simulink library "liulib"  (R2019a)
settings: Solver=ode45  StartTime=0.0  StopTime=10.0  RelTol=1e-3  EnableMultiTasking=on
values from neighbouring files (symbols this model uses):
  ag = ones(ng,1); [fPg,fTg] = bfgenD(0,P)    [bfgenD.m]    (also in fbtfit.m = AA \ [Ip ; rBt^2 ; 0]; fbtt.m = zeros(L.ng,1); fgeFpicard.m = x(2+(1:L.ng)))
  aq = []    [fbtt.m]
  aW = []    [fbtt.m]
  D = Fyi1j + Fyim1j + A.*Fyij1  +B.*Fyijm1 - C.*Fyij    [dlst.m]    (also in fbtp.m = meqp(); fgep.m = fgsp(P,varargin{:}))
  dr2FA = dr2Fs(1:nA,1)    [asxycs.m]
  drzFA = drzFs(1:nA,1)    [asxycs.m]
  dz = (z - zx(kz))/dzx    [bintc.m]
  dz2FA = dz2Fs(1:nA,1)    [asxycs.m]
  FA = Fs(1:nA,1)    [asxycs.m]    (also in bfhelp.m = [-1                        0      	 0])
  FB = [0                         1        1]    [bfhelp.m]
  Fx = zeros(n+2,3); Fx(2:end-1,2) = FN    [bfhelp.m]    (also in fbtt.m = meqFx(L,Iy,[Ia;Iu]); fgeFpicard.m = FxP + Fxe)
  FX = Fs(nA+1:ns,1)    [asxycs.m]
  Ie = [Ia;Iu]    [fgeF.m]    (also in fgeFpicard.m = (L.Mee + diag(LXt.dt*L.Re))\       ([LXt.dt*LXt.Va;zeros(L.G)
  IpD = LX.IpD(:,kt)    [fbtt.m]    (also in fgeFpicard.m = LXt.(L.agconc{1,3}))
  Iy = (Iy+flipud(Iy))*0.5    [fbtt.m]    (also in fgeF.m = reshape( xnl(L.ind.iy) , L.nzy, L.nry); fgeFpicard.m = Iyscal*reshape(Tyg*ag,L.nzy,L.nry))
  L = fbtc(P,G)    [fbt.m]    (also in fbtc.m = meqc(P,G,'rrx','zzx'); fbte.m = varargout{1}; fge.m = fgel(L,meqxk(LX,1)); fgec.m = fgsc(P,G))
  lB = false    [fbtt.m]
  lX = false    [fbtt.m]
  nA = numel(rA)    [asxycs.m]    (also in fbtt.m; fgeFpicard.m)
  niter = L.P.itercs    [asxycs.m]    (also in fbtt.m = 2)
  Opy = zeros(meqsize(L, 'Opy'),'int8')    [fbtt.m]
  rA = rs(1:nA,1)    [asxycs.m]    (also in fbtptcv.m = (rA1 + 3*rA2)/4)
  rBt = LX.rBt(kt)    [fbtt.m]    (also in fgeFpicard.m = LXt.rBt)
  rX = rs(nA+1:ns,1)    [asxycs.m]    (also in fbtptcv.m = rzbro(iX,1); fbtxana.m = r0 + [1; 1]*a0*0.5)
  zA = zs(1:nA,1)    [asxycs.m]    (also in fbtptcv.m = (zA1 + 3*zA2)/4)
  zX = zs(nA+1:ns,1)    [asxycs.m]    (also in fbtptcv.m = rzbro(iX,2); fbtxana.m = z0 + [1;-1]*a0*1.0)
undefined symbols (not defined in the file or in its folder): aminor, Bm, bp, bpli2, Brn, Brrn, Brzn, bt, Bzn, Bzrn, Bzzn, delta, deltal, deltau, dzg, epsilon, err, Ff, Fn, Ft, Ft0, FW, Ip, iqQ, iTQ, jtorQ, kappa, li, lp, mu, nX, PpQ, PQ, Q0Q, Q1Q, Q2Q, Q3Q, Q4Q, q95, qmin, raQ, raqmin, rB, rbary, repmat, rgeom, rIp, rIpD, Row, rq, rS, rst, TQ, TTpQ, vector, Vn, Vp, Wk, WN, Wp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
libraries: $bdroot x52, mkllib x48, simulink x7
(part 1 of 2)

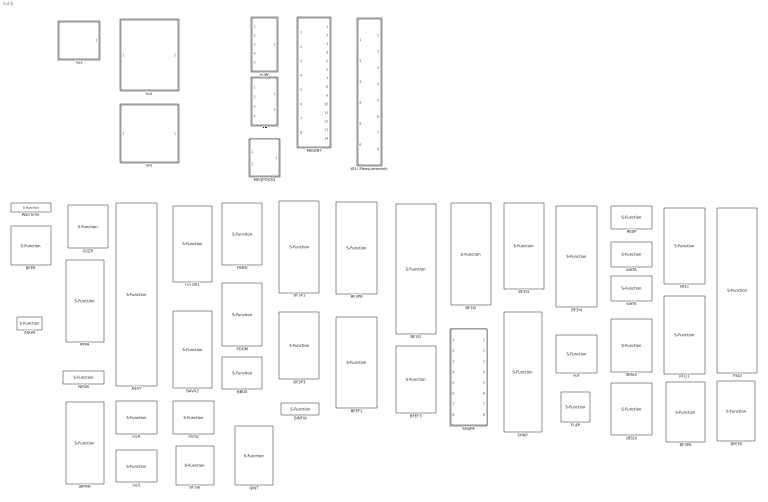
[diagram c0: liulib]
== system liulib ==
  ASGN : S-Function  FunctionName=sasgncsf  Parameters=iu  SFunctionDeploymentMode=off  EnableBusSupport=off  mask{iu=0}
  ASXY : S-Function  FunctionName=sasxycsf  Parameters=rx zx dr dz idr idz Oasx daxm  SFunctionDeploymentMode=off  EnableBusSupport=off  mask{rx=L.G.rx, zx=L.G.zx, dr=L.drx, dz=L.dzx, idr=L.idrx, idz=L.idzx, Oasx=L.Oasx, daxm=L.P.daxm}
      mask prompts: rx "rx [28]"; zx "zx [65]"
      mask help: Axis and Saddle point finder on xy grid
  BAVX2 : S-Function  FunctionName=sbavx2csf  Parameters=a  SFunctionDeploymentMode=off  EnableBusSupport=off  mask{a=0}
      mask prompts: a "alpha"
  BBOX : S-Function  FunctionName=sbboxcsf  Parameters=z r  SFunctionDeploymentMode=off  EnableBusSupport=off  mask{z=L.zy, r=L.ry}
  BF3I1 : S-Function  FunctionName=sbf3i1csf  Parameters=r ir nz nr  SFunctionDeploymentMode=off  EnableBusSupport=off  mask{r=L.ry, ir=L.iry, nz=L.nzy, nr=L.nry}
      mask prompts: r "r inner grid"; ir "ir inner grid"; nz "nzy"; nr "nry"
  BF3I2 : S-Function  FunctionName=sbf3i2csf  SFunctionDeploymentMode=off  EnableBusSupport=off
  BF3I3 : S-Function  FunctionName=sbf3i3csf  Parameters=idsx  SFunctionDeploymentMode=off  EnableBusSupport=off  mask{idsx=L.idsx}
  BF3I4 : S-Function  FunctionName=sbf3i4csf  Parameters=nzy nry  SFunctionDeploymentMode=off  EnableBusSupport=off  mask{nzy=L.nzy, nry=L.nry}
  BF3I6 : S-Function  FunctionName=sbf3i6csf  SFunctionDeploymentMode=off  EnableBusSupport=off
  BF3P1 : S-Function  FunctionName=sbf3p1csf  Parameters=ry iry nzy nry  SFunctionDeploymentMode=off  EnableBusSupport=off  mask{ry=L.ry, iry=L.iry, nzy=L.nzy, nry=L.nry}
      mask prompts: ry "ry inner grid"; iry "iry inner grid"
  BF3P3 : S-Function  FunctionName=sbf3p3csf  Parameters=idsx  SFunctionDeploymentMode=off  EnableBusSupport=off  mask{idsx=L.idsx}
  BF3P6 : S-Function  FunctionName=sbf3p6csf  SFunctionDeploymentMode=off  EnableBusSupport=off
  BF3P8 : S-Function  FunctionName=sbf3p8csf  Parameters=ids iry  SFunctionDeploymentMode=off  EnableBusSupport=off  mask{ids=L.idsx, iry=L.iry}
      mask prompts: ids "r inner grid"; iry "ir inner grid"
  BFEF1 : S-Function  FunctionName=sbfef1csf  Parameters=ry iry nzy nry nP nT  SFunctionDeploymentMode=off  EnableBusSupport=off  mask{ry=L.ry, iry=L.iry, nzy=L.nzy, nry=L.nry, nP=L.P.bfp(1), nT=L.P.bfp(2)}
      mask prompts: ry "ry inner grid"; iry "iry inner grid"
  BFEF3 : S-Function  FunctionName=sbfef3csf  Parameters=ids nP nT  SFunctionDeploymentMode=off  EnableBusSupport=off  mask{ids=L.idsx, nP=L.P.bfp(1), nT=L.P.bfp(2)}
  BFEF6 : S-Function  FunctionName=sbfef6csf  Parameters=nP nT nq  SFunctionDeploymentMode=off  EnableBusSupport=off  mask{nP=L.P.bfp(1), nT=L.P.bfp(2), nq=L.nq}
  BFPR : S-Function  FunctionName=sbfprcsf  SFunctionDeploymentMode=off  EnableBusSupport=off
  BINTW : S-Function  FunctionName=sbintcsf  Parameters=kxW cWx nzx  SFunctionDeploymentMode=off  EnableBusSupport=off  mask{kxW=L.kxW, cWx=L.cWx, nzx=L.nzx}
  FBND : S-Function  FunctionName=sfbndcsf  Parameters=rl zl  SFunctionDeploymentMode=off  EnableBusSupport=off  mask{rl=L.G.rl, zl=L.G.zl}
  FE : Subsystem  Variant=on
  FL4P : S-Function  FunctionName=sfl4pcsf  Parameters=kl cl nz  SFunctionDeploymentMode=off  EnableBusSupport=off  mask{kl=int32(L.kxl-1), cl=L.clx, nz=L.nzx}
      mask prompts: kl "kl 0-based"; cl "cl [4][]"
  FSGI : S-Function  FunctionName=sfsgicsf  Parameters=idoq  SFunctionDeploymentMode=off  EnableBusSupport=off  mask{idoq=1/L.doq}
      mask help: Flux Surface Geometric Integrals
  GSZR : S-Function  FunctionName=sgszrcsf  Parameters=cx cq cr cs ci co  SFunctionDeploymentMode=off  EnableBusSupport=off  mask{cx=L.cx, cq=L.cq, cr=L.cr, cs=L.cs, ci=L.ci, co=L.co}
      mask help: Grad-Shafranov equation on RZ grid
  IPMH : S-Function  FunctionName=sipmhcsf  Parameters=Ahd Aed Ahe Aeh Ahh uAhh nit  SFunctionDeploymentMode=off  EnableBusSupport=off  mask{Ahd=L.Ahd, Aed=L.Aed, Ahe=L.Ahe, Aeh=L.Aeh, Ahh=L.Ahh, uAhh=L.uAhh, nit=L.P.iterh}
      mask prompts: nit "Maximum iteration #"
  MEQINT : Subsystem
  MEQPOSTQ : Subsystem  TreatAsAtomicUnit=on  VariantControl=liuITERQMODEvariant1
  NFDB : S-Function  FunctionName=snfdbcsf  Parameters=nz nr  SFunctionDeploymentMode=off  EnableBusSupport=off  mask{nz=L.nzx, nr=L.nrx}
  PDOM : S-Function  FunctionName=spdomcsf  SFunctionDeploymentMode=off  EnableBusSupport=off
      mask help: Plasma DOmain finder
  QINT : S-Function  FunctionName=sqintcsf  Parameters=rx zx inM  SFunctionDeploymentMode=off  EnableBusSupport=off  mask{rx=L.rx, zx=L.zx, inM=L.inM}
  RESP : S-Function  FunctionName=srespcsf  Parameters=A B nr ng  SFunctionDeploymentMode=off  EnableBusSupport=off  mask{A=L.Wr.*L.Mry, B=L.P.fdz*(L.Wr.*L.Mdzry), nr=L.nr, ng=L.ng}
      mask prompts: A "Mry"; B "Mdzry"
  RTCI : S-Function  FunctionName=srtcicsf  Parameters=c s da nr nz  SFunctionDeploymentMode=off  EnableBusSupport=off  mask{c=L.cdrq, s=L.cdzq, da=L.drx, nr=L.nrx, nz=L.nzx}
      mask prompts: c "cos(theta)*dr"; s "sin(theta)*dz"; da "delta a max"
      mask help: Real-Time Contour Integration
  RTCI1 : S-Function  FunctionName=srtci1csf  SFunctionDeploymentMode=off  EnableBusSupport=off
  SHAP : S-Function  FunctionName=sshapcsf  Parameters=dr dz npq noq  SFunctionDeploymentMode=off  EnableBusSupport=off  mask(Computes shape parameters from rq,zq contours){dr=L.drx, dz=L.dzx, npq=L.npq, noq=L.noq}
      mask help: See shapmex.c, shap.c
  SHAPE : Subsystem  mask(meqshape){dr=L.drx, dz=L.dzx, npq=L.npq, noq=L.noq}
      mask help: Calculates LCFS shape information. See meqshape.m for details
  Wall time : S-Function  FunctionName=swclkcsf  Parameters=f  SFunctionDeploymentMode=off  EnableBusSupport=off  mask{f=1e6}
      mask prompts: f "Factor (e.g. 1000 for ms)"
  dBSLV : S-Function  FunctionName=dbslvcsf  Parameters=niter  SFunctionDeploymentMode=off  EnableBusSupport=off  mask{niter=L.P.iters}
  dIATA : S-Function  FunctionName=diatacsf  SFunctionDeploymentMode=off  EnableBusSupport=off
  dIPMH : S-Function  FunctionName=dipmhcsf  Parameters=Ahd Aed Ahe Aeh Ahh uAhh nit  SFunctionDeploymentMode=off  EnableBusSupport=off  mask{Ahd=0, Aed=0, Ahe=0, Aeh=0, Ahh=0, uAhh=0, nit=0}
      mask prompts: nit "Maximum iteration #"
  l in OX1 : S-Function  FunctionName=sbavxcsf  Parameters=a  SFunctionDeploymentMode=off  EnableBusSupport=off  mask{a=0}
      mask prompts: a "alpha"
  liht : Subsystem  TreatAsAtomicUnit=on
  liuW : Subsystem  TreatAsAtomicUnit=on
  liut : Subsystem  TreatAsAtomicUnit=on
  liux : Subsystem
  locR : S-Function  FunctionName=slocRcsf  Parameters=nR naR  SFunctionDeploymentMode=off  EnableBusSupport=off  mask{nR=numel(L.P.iqR), naR=1}
  locS : S-Function  FunctionName=slocScsf  SFunctionDeploymentMode=off  EnableBusSupport=off
  minQ : S-Function  FunctionName=sminQcsf  Parameters=nmin  SFunctionDeploymentMode=off  EnableBusSupport=off  mask{nmin=1}
  sBSLV : S-Function  FunctionName=sbslvcsf  Parameters=niter  SFunctionDeploymentMode=off  EnableBusSupport=off  mask{niter=L.P.iters}
  sIATA : S-Function  FunctionName=siatacsf  SFunctionDeploymentMode=off  EnableBusSupport=off
  t01/ Measurements : Subsystem
  vizr : S-Function  FunctionName=svizrcsf  Parameters=ry iry dr dz nr nz  SFunctionDeploymentMode=off  EnableBusSupport=off  mask{ry=L.ry, iry=L.iry, dr=L.drx, dz=L.dzx, nr=L.nrx, nz=L.nzx}
      mask prompts: ry "r inner grid"; iry "ir inner grid"

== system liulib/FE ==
  Yd : Inport
  Ie : Inport  Port=2
  Ip : Inport  Port=3
  sIp : Inport  Port=4
  FE ipm : Subsystem  VariantControl=liuHFCTMODEvariant2
  FE ipm double : Subsystem  VariantControl=liuHFCTMODEvariant3
  FE lsq : Subsystem  VariantControl=liuHFCTMODEvariant1
  Jh : Outport
  Je : Outport  Port=2

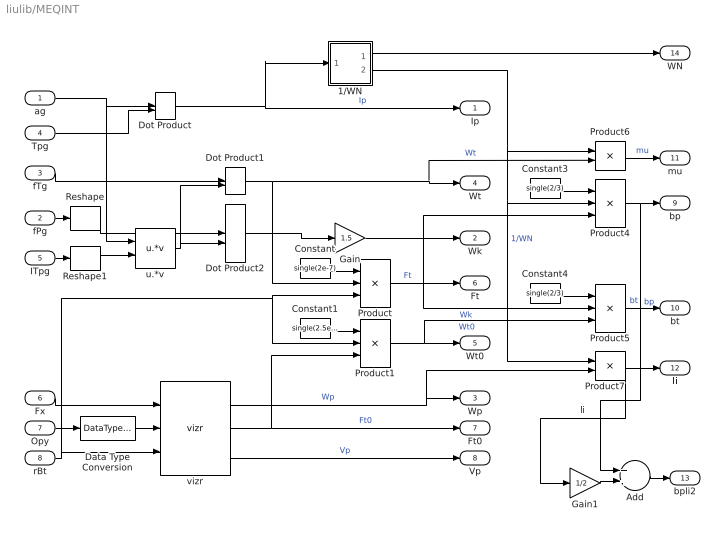
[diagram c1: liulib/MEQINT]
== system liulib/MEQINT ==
  ag : Inport
  fPg : Inport  Port=2
  fTg : Inport  Port=3
  Tpg : Inport  Port=4
  ITpg : Inport  Port=5
  Fx : Inport  Port=6
  Opy : Inport  Port=7
  rBt : Inport  Port=8
  1/WN : Subsystem
  Add : Sum
  Constant : Constant  Value=single(2e-7)  OutDataTypeStr=single
  Constant1 : Constant  Value=single(2.5e6)  OutDataTypeStr=single
  Constant3 : Constant  Value=single(2/3)  OutDataTypeStr=single
  Constant4 : Constant  Value=single(2/3)  OutDataTypeStr=single
  Data Type Conversion : DataTypeConversion  OutDataTypeStr=boolean
  Dot Product : DotProduct
  Dot Product1 : DotProduct
  Dot Product2 : DotProduct
  Gain : Gain  Gain=1.5
  Gain1 : Gain  Gain=1/2
  Product : Product  Inputs=**/
  Product1 : Product  Inputs=3
  Product4 : Product  Inputs=3
  Product5 : Product  Inputs=**/
  Product6 : Product
  Product7 : Product
  Reshape : Reshape
  Reshape1 : Reshape
  u.*v : mkllib/u.*v
  vizr : $bdroot/vizr  ry=L.ry  iry=L.iry  dr=L.drx  dz=L.dzx  nr=L.nrx  nz=L.nzx
  Ip : Outport
  Wk : Outport  Port=2
  Wp : Outport  Port=3
  Wt : Outport  Port=4
  Wt0 : Outport  Port=5
  Ft : Outport  Port=6
  Ft0 : Outport  Port=7
  Vp : Outport  Port=8
  bp : Outport  Port=9
  bt : Outport  Port=10
  mu : Outport  Port=11
  li : Outport  Port=12
  bpli2 : Outport  Port=13
  WN : Outport  Port=14
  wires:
  1/WN/1(WN) -> WN/1
  Gain1/1 -> Add/2
  Add/1 -> bpli2/1
  vizr/3 -> Vp/1  "Vp"
  Fx/1 -> vizr/1
  rBt/1 -> Product1/2, Product/3, vizr/3
  ag/1 -> u.*v/1, Dot Product/1
  Tpg/1 -> Dot Product/2
  u.*v/1 -> Dot Product1/2, Dot Product2/2
  Dot Product/1 -> 1/WN/1(Ip), Ip/1  "Ip"
  Dot Product2/1 -> Gain/1
  vizr/1 -> Product7/2, Wp/1  "Wp"
  Dot Product1/1 -> Product/2, Product6/2, Wt/1  "Wt"
  fTg/1 -> Dot Product1/1
  vizr/2 -> Ft0/1, Product1/3  "Ft0"
  Constant/1 -> Product/1
  Product/1 -> Ft/1  "Ft"
  Constant1/1 -> Product1/1
  Product1/1 -> Product5/3, Wt0/1  "Wt0"
  Constant3/1 -> Product4/1
  Product4/1 -> bp/1, Add/1  "bp"
  Product5/1 -> bt/1  "bt"
  Constant4/1 -> Product5/1
  Product6/1 -> mu/1  "mu"
  Product7/1 -> li/1, Gain1/1  "li"
  Gain/1 -> Product5/2, Product4/3, Wk/1  "Wk"
  1/WN/2(1/WN) -> Product6/1, Product7/1, Product4/2  "1/WN"
  fPg/1 -> Reshape/1
  ITpg/1 -> Reshape1/1
  Reshape/1 -> Dot Product2/1
  Reshape1/1 -> u.*v/2
  Opy/1 -> Data Type Conversion/1
  Data Type Conversion/1 -> vizr/2

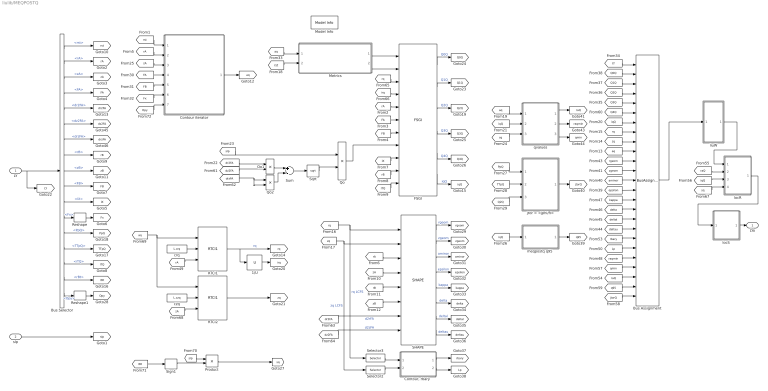
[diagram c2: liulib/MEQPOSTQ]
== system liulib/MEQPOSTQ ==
  LY : Inport
  sIp : Inport  Port=2
  1/U : mkllib/1//U
  Bus Assignment : BusAssignment  AssignedSignals=Q0Q,Q1Q,Q2Q,Q3Q,Q4Q,iqQ,rq,zq,aq,rgeom,zgeom,aminor,epsilon,kappa,delta,deltal,deltau,rbary,lp,raqmin,qmin,raQ,q95,jtorQ
  Bus Selector : BusSelector  OutputSignals=rst,rA,zA,FA,dr2FA,dz2FA,drzFA,rB,zB,FB,lX,Fx,PpQ,TTpQ,iTQ,rBt,Opy
  Contour iterator : Subsystem
  "Contour, rbary " : Subsystem
  FSGI : $bdroot/FSGI  idoq=1/L.doq
  Metrics : Subsystem
  Model Info : simulink/Model-Wide Utilities/Model Info  Frame=on  DisplayStringWithTags=|  HorizontalTextAlignment=Center  LeftAlignmentValue=0.5
      | Model Info
      | %<Creator>
      | %<ModifiedBy>
      | %<ModifiedDate>
      | %<ModifiedComment>
      | %<ModelVersion>
  Product : Product
  Qo : Product  Inputs=**
  Qo1 : Product  Inputs=**
  Qo2 : Product  Inputs=**
  RTCI1 : $bdroot/RTCI1  SFunctionModules=''
  RTCI2 : $bdroot/RTCI1  SFunctionModules=''
  Reshape : Reshape  OutputDimensions=L.nzx*L.nrx
  Reshape1 : Reshape  OutputDimensions=L.nzy*L.nry
  SHAPE : $bdroot/SHAPE  dr=L.drx  dz=L.dzx  npq=L.npq  noq=L.noq
  Selector2 : Selector  NumberOfDimensions=2  InputPortWidth=3  IndexOptions=Select all,Index vector (dialog)  Indices=[1 3],L.npq  OutputSizes=1,1
  Selector3 : Selector  NumberOfDimensions=2  InputPortWidth=3  IndexOptions=Select all,Index vector (dialog)  Indices=[1 3],L.npq  OutputSizes=1,1
  Sign1 : Signum
  Sqrt : Sqrt
  Sum : Sum  Inputs=+-
  crq : Constant  Value=L.crq  OutDataTypeStr=single
  czq : Constant  Value=L.czq  OutDataTypeStr=single
  jtor = <jphi/R> : Subsystem
  liuW : Subsystem  Variant=on  VariantControl=Variant1
  locR : Subsystem  Variant=on  VariantControl=Variant1
  locS : Subsystem  Variant=on  VariantControl=Variant1
  "meqpostq q95 " : Subsystem
  qvalues : Subsystem
  LYo : Outport
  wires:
  "Contour, rbary "/1(rbary) -> [rbary]
  "Contour, rbary "/2(Lp) -> [Lp]
  qvalues/2(raqmin) -> [raqmin]
  qvalues/3(qmin) -> [qmin]
  [iTQ] -> FSGI/11
  FSGI/1 -> [Q0Q]  "Q0Q"
  Bus Selector/5 -> [dr2FA]  "<dr2FA>"
  SHAPE/3 -> [aminor]  "aminor"
  Bus Selector/4 -> [FA]  "<FA>"
  SHAPE/1 -> [rgeom]  "rgeom"
  SHAPE/8 -> [deltau]  "deltau"
  [rq] -> SHAPE/1, Selector3/1  "rq LCFS"
  [sIp] -> Qo/1
  [iqQ] -> qvalues/2(iqQ)
  Selector2/1 -> "Contour, rbary "/2(zq)
  Bus Selector/2 -> [rA]  "<rA>"
  SHAPE/6 -> [delta]  "delta"
  [rB] -> FSGI/10
  Bus Selector/3 -> [zA]  "<zA>"
  FSGI/4 -> [Q3Q]  "Q3Q"
  Sum/1 -> Sqrt/1
  [zq] -> SHAPE/2, Selector2/1  "zq LCFS"
  [FB] -> FSGI/7
  Metrics/1(da^2/pdp = M1q) -> FSGI/1
  FSGI/6 -> [iqQ]  "iqQ"
  Sqrt/1 -> Qo/2
  [dz2FA] -> SHAPE/8  "d2zFA"
  [sq] -> qvalues/3(sq)
  [aq] -> qvalues/1(aq)
  [dr2FA] -> Qo1/1
  [rst] -> Metrics/2(rst)
  [rB] -> SHAPE/5
  FSGI/2 -> [Q1Q]  "Q1Q"
  [zA] -> SHAPE/4
  Qo1/1 -> Sum/1
  Selector3/1 -> "Contour, rbary "/1(rq)
  SHAPE/4 -> [epsilon]  "epsilon"
  SHAPE/2 -> [zgeom]  "zgeom"
  SHAPE/7 -> [deltal]  "deltal"
  [drzFA] -> Qo2/2, Qo2/1
  [rA] -> SHAPE/3
  [rA] -> FSGI/5
  Qo/1 -> FSGI/8
  [FA] -> FSGI/6
  Qo2/1 -> Sum/2
  Metrics/2(((da^2/2do)^2+a^2)/(da^2/pdp) = M2q) -> FSGI/2
  [zB] -> SHAPE/6
  [lX] -> FSGI/9
  [dr2FA] -> SHAPE/7  "d2rFA"
  SHAPE/5 -> [kappa]  "kappa"
  [dz2FA] -> Qo1/2
  sIp/1 -> [sIp]
  FSGI/3 -> [Q2Q]  "Q2Q"
  FSGI/5 -> [Q4Q]  "Q4Q"
  Bus Selector/1 -> [rst]  "<rst>"
  [iqQ] -> "meqpostq q95 "/1(iqQ)
  "meqpostq q95 "/1(q95) -> [q95]
  [PpQ] -> jtor = <jphi/R>/1(PpQ)
  [TTpQ] -> jtor = <jphi/R>/2(TTpQ)
  [Q2Q] -> jtor = <jphi/R>/3(Q2Q)
  jtor = <jphi/R>/1(jtorQ) -> [jtorQ]
  qvalues/1(raQ) -> [raQ]
  [zA] -> Contour iterator/3(zA)
  [FB] -> Contour iterator/5(FB)
  [rst] -> Contour iterator/1(rst)
  [rA] -> Contour iterator/2(rA)
  [FA] -> Contour iterator/4(FA)
  [Fx] -> Contour iterator/6(Fx)
  Contour iterator/1(aq) -> [aq]
  [aq] -> Metrics/1(aq)
  LY/1 -> [LY], Bus Selector/1
  [jtorQ] -> Bus Assignment/25
  [q95] -> Bus Assignment/24
  [Lp] -> Bus Assignment/20
  [rbary] -> Bus Assignment/19
  [deltau] -> Bus Assignment/18
  [deltal] -> Bus Assignment/17
  [delta] -> Bus Assignment/16
  [kappa] -> Bus Assignment/15
  [epsilon] -> Bus Assignment/14
  [aminor] -> Bus Assignment/13
  [zgeom] -> Bus Assignment/12
  [rgeom] -> Bus Assignment/11
  [aq] -> Bus Assignment/10
  [zq] -> Bus Assignment/9
  [rq] -> Bus Assignment/8
  [iqQ] -> Bus Assignment/7
  [Q4Q] -> Bus Assignment/6
  [Q3Q] -> Bus Assignment/5
  [Q2Q] -> Bus Assignment/4
  [Q1Q] -> Bus Assignment/3
  [Q0Q] -> Bus Assignment/2
  [LY] -> Bus Assignment/1
  Bus Selector/6 -> [dz2FA]  "<dz2FA>"
  Bus Selector/7 -> [drzFA]  "<drzFA>"
  Bus Selector/8 -> [rB]  "<rB>"
  Bus Selector/9 -> [zB]  "<zB>"
  Bus Selector/10 -> [FB]  "<FB>"
  Bus Selector/11 -> [lX]  "<lX>"
  Bus Selector/13 -> [PpQ]  "<PpQ>"
  Bus Selector/14 -> [TTpQ]  "<TTpQ>"
  Bus Selector/15 -> [iTQ]  "<iTQ>"
  Reshape/1 -> [Fx]
  Bus Selector/12 -> Reshape/1  "<Fx>"
  [irq] -> FSGI/4
  [rq] -> FSGI/3
  locS/1(" LYo") -> LYo/1
  Bus Assignment/1 -> liuW/1(LY)
  [raQ] -> locR/2("raQ ")
  [iqQ] -> locR/3("qQ ")
  [sq] -> locR/4(sq)
  liuW/1(LYo) -> locR/1(LY)
  locR/1(" LYo") -> locS/1("LY ")
  [raqmin] -> Bus Assignment/21
  [qmin] -> Bus Assignment/22
  [raQ] -> Bus Assignment/23
  RTCI1/1 -> [rq], 1/U/1  "rq"
  crq/1 -> RTCI1/2
  czq/1 -> RTCI2/2
  [zA] -> RTCI2/3
  [aq] -> RTCI2/1, RTCI1/1
  [rA] -> RTCI1/3
  1/U/1 -> [irq]
  RTCI2/1 -> [zq]
  Sign1/1 -> Product/2
  [sIp] -> Product/1
  Product/1 -> [sq]
  Bus Selector/16 -> [rBt]  "<rBt>"
  [rBt] -> Sign1/1
  [Opy] -> Contour iterator/7(Opy)
  Bus Selector/17 -> Reshape1/1  "<Opy>"
  Reshape1/1 -> [Opy]

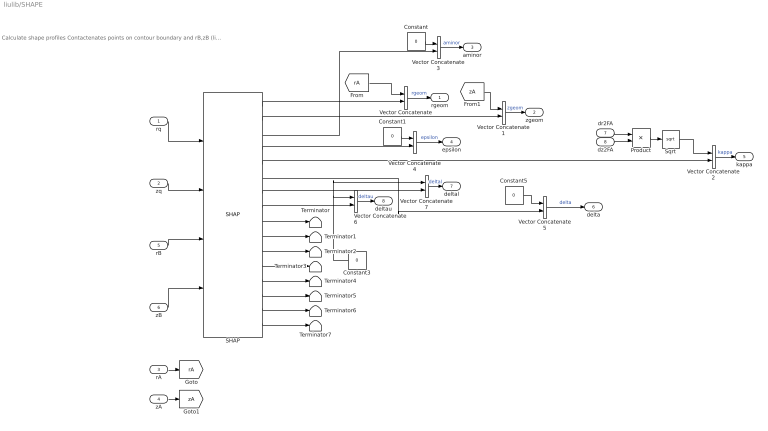
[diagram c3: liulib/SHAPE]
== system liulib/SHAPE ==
  note: Calculate shape profiles Contactenates points on contour boundary and rB,zB (limiter/divertor point) see also meqshape.m
  rq : Inport  OutDataTypeStr=single
  zq : Inport  Port=2  OutDataTypeStr=single
  rA : Inport  Port=3  OutDataTypeStr=single
  zA : Inport  Port=4  OutDataTypeStr=single
  rB : Inport  Port=5  OutDataTypeStr=single
  zB : Inport  Port=6  OutDataTypeStr=single
  dr2FA : Inport  Port=7
  dz2FA : Inport  Port=8
  Constant{,1,3,5} (4 alike) : Constant  Value=0  OutDataTypeStr=single
  Product : Product  Inputs=*/
  SHAP : $bdroot/SHAP  dr=L.drx  dz=L.dzx  npq=L.npq  noq=L.noq
  Sqrt : Sqrt
  Terminator{,1..7} (8 alike) : Terminator
  Vector Concatenate{,1..7} (8 alike) : Concatenate
  rgeom : Outport
  zgeom : Outport  Port=2
  aminor : Outport  Port=3
  epsilon : Outport  Port=4
  kappa : Outport  Port=5
  delta : Outport  Port=6
  deltal : Outport  Port=7
  deltau : Outport  Port=8
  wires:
  SHAP/6 -> Vector Concatenate5/2
  SHAP/4 -> Vector Concatenate4/2
  rq/1 -> SHAP/1
  zq/1 -> SHAP/2
  zB/1 -> SHAP/4
  rB/1 -> SHAP/3
  SHAP/1 -> Vector Concatenate/2
  SHAP/3 -> Vector Concatenate3/2
  SHAP/5 -> Vector Concatenate2/2
  SHAP/7 -> Vector Concatenate7/2
  SHAP/9 -> Terminator/1
  SHAP/8 -> Vector Concatenate6/2
  SHAP/10 -> Terminator1/1
  SHAP/11 -> Terminator2/1
  SHAP/12 -> Terminator3/1
  SHAP/13 -> Terminator4/1
  SHAP/14 -> Terminator5/1
  SHAP/15 -> Terminator6/1
  SHAP/16 -> Terminator7/1
  Vector Concatenate/1 -> rgeom/1  "rgeom"
  rA/1 -> [rA]
  [rA] -> Vector Concatenate/1
  zA/1 -> [zA]
  [zA] -> Vector Concatenate1/1
  SHAP/2 -> Vector Concatenate1/2
  Vector Concatenate1/1 -> zgeom/1  "zgeom"
  Vector Concatenate2/1 -> kappa/1  "kappa"
  Vector Concatenate3/1 -> aminor/1  "aminor"
  Vector Concatenate4/1 -> epsilon/1  "epsilon"
  Constant/1 -> Vector Concatenate3/1
  Constant1/1 -> Vector Concatenate4/1
  Vector Concatenate5/1 -> delta/1  "delta"
  Vector Concatenate6/1 -> deltau/1  "deltau"
  Constant3/1 -> Vector Concatenate7/1, Vector Concatenate6/1
  Vector Concatenate7/1 -> deltal/1  "deltal"
  Constant5/1 -> Vector Concatenate5/1
  Product/1 -> Sqrt/1
  Sqrt/1 -> Vector Concatenate2/1
  dz2FA/1 -> Product/2
  dr2FA/1 -> Product/1

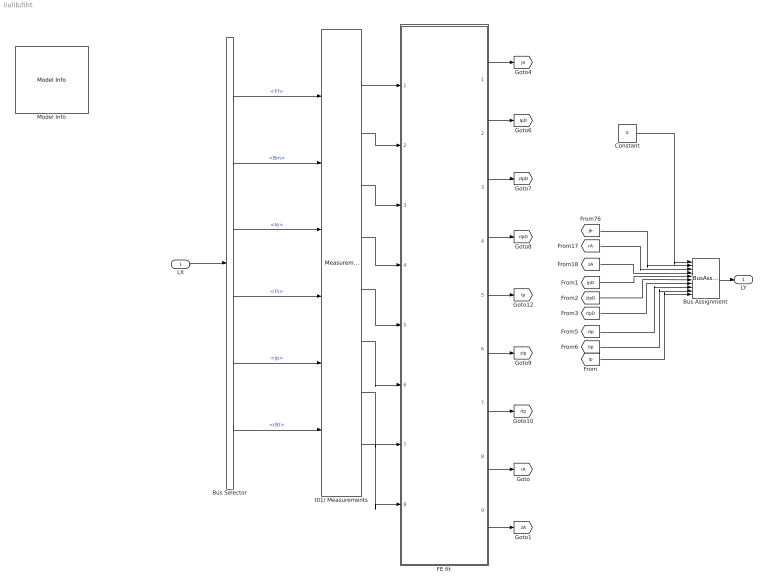
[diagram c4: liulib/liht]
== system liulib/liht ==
  LX : Inport
  Bus Assignment : BusAssignment  AssignedSignals=Ie,rA,zA,IpD,zIpD,rIpD,zIp,rIp,Ip
  Bus Selector : BusSelector  OutputSignals=Ff,Bm,Ie,Ft,Ip,rBt
  Constant : Constant  Value=0  OutDataTypeStr=Bus: LYbus
  FE fit : Subsystem
  Model Info : simulink/Model-Wide Utilities/Model Info  Frame=on  DisplayStringWithTags=|  HorizontalTextAlignment=Center  LeftAlignmentValue=0.5
      | Model Info
      | %<Creator>
      | %<ModifiedBy>
      | %<ModifiedDate>
      | %<ModifiedComment>
      | %<ModelVersion>
  t01/ Measurements : $bdroot/t01// Measurements  SystemSampleTime=-1
  LY : Outport
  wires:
  FE fit/6(Out7) -> [zIp]
  FE fit/7(Out8) -> [rIp]
  FE fit/5(Out9) -> [Ip]
  FE fit/8(Out5) -> [rA]
  [Ip] -> Bus Assignment/10
  [rIp] -> Bus Assignment/9
  [zIp] -> Bus Assignment/8
  Bus Assignment/1 -> LY/1
  Bus Selector/6 -> t01/ Measurements/6  "<rBt>"
  Bus Selector/4 -> t01/ Measurements/4  "<Ft>"
  t01/ Measurements/4 -> FE fit/4(Ie)
  Bus Selector/3 -> t01/ Measurements/3  "<Ie>"
  Bus Selector/5 -> t01/ Measurements/5  "<Ip>"
  LX/1 -> Bus Selector/1
  t01/ Measurements/8 -> FE fit/8(sIp)
  t01/ Measurements/7 -> FE fit/7(FN)
  t01/ Measurements/6 -> FE fit/6(rBt)
  t01/ Measurements/5 -> FE fit/5(Ip)
  t01/ Measurements/3 -> FE fit/3(Yi)
  t01/ Measurements/2 -> FE fit/2(Yd)
  Bus Selector/1 -> t01/ Measurements/1  "<Ff>"
  Bus Selector/2 -> t01/ Measurements/2  "<Bm>"
  t01/ Measurements/1 -> FE fit/1(Yr)
  FE fit/1(Out4) -> [Je]
  FE fit/9(Out6) -> [zA]
  FE fit/2(Out1) -> [IpD]
  FE fit/3(Out2) -> [zIpD]
  FE fit/4(Out3) -> [rIpD]
  Constant/1 -> Bus Assignment/1
  [Je] -> Bus Assignment/2
  [IpD] -> Bus Assignment/5
  [zIpD] -> Bus Assignment/6
  [rIpD] -> Bus Assignment/7
  [rA] -> Bus Assignment/3
  [zA] -> Bus Assignment/4

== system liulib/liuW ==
  zaW : Inport
  rst : Inport  Port=2
  FW : Inport  Port=3
  Fx : Inport  Port=4
  Opy : Inport  Port=5
  BINTW : $bdroot/BINTW  kxW=L.kxW  cWx=L.cWx  nzx=L.nzx
  Constant : Constant  Value=int8(0)
  IC = 1 : UnitDelay  InitialCondition=1  SampleTime=-1  HasFrameUpgradeWarning=on
  RTCI : $bdroot/RTCI  c=L.cdrW  s=L.cdzW  da=L.drx  nr=L.nrx  nz=L.nzx
  Reshape1 : Reshape
  Reshape2 : Reshape
  "aq " : Switch  Criteria=u2 ~= 0
  dan : Terminator
  rx1 : Constant  Value=L.erW  OutDataTypeStr=single
  rx2 : Constant  Value=L.ezW  OutDataTypeStr=single
  rx3 : Constant  Value=zeros(L.G.nW,L.P.nFW)  VectorParams1D=off  OutDataTypeStr=single
  aW : Outport
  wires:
  Reshape2/1 -> RTCI/6
  Reshape1/1 -> BINTW/1, RTCI/4
  rst/1 -> IC = 1/1
  zaW/1 -> "aq "/3
  FW/1 -> RTCI/5
  "aq "/1 -> RTCI/1
  RTCI/2 -> dan/1
  rx1/1 -> RTCI/2
  rx2/1 -> RTCI/3
  Fx/1 -> Reshape1/1
  rx3/1 -> "aq "/1
  RTCI/1 -> aW/1  "aW"
  BINTW/1 -> RTCI/7
  Constant/1 -> RTCI/8
  Opy/1 -> Reshape2/1
  IC = 1/1 -> "aq "/2

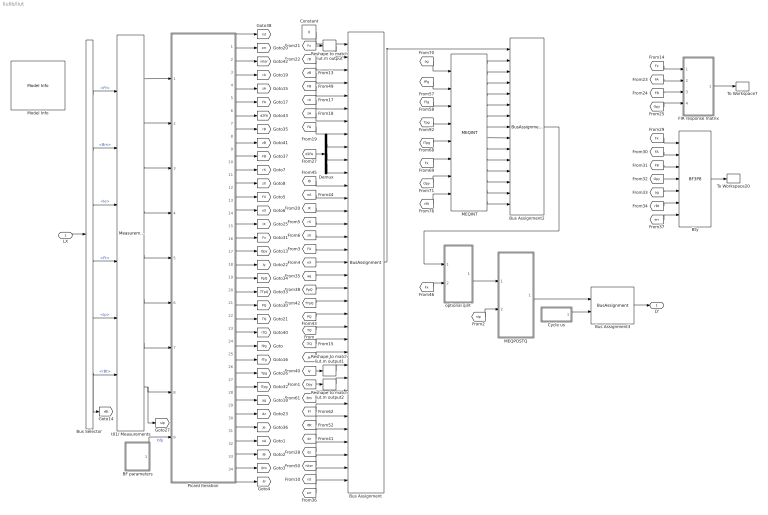
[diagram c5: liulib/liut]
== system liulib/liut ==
  LX : Inport
  BF parameters : Subsystem  Variant=on  VariantControl=Variant1
  Bty : $bdroot/BF3P8  Commented=on  ids=L.idsx  iry=L.iry
  Bus Assignment : BusAssignment  AssignedSignals=Fx,rB,zB,FB,rA,zA,FA,dr2FA,dz2FA,drzFA,lB,nA,lX,rX,zX,FX,nX,ag,PpQ,TTpQ,PQ,TQ,iTQ,Ie,Iy,Opy,Bm,Ff,rBt,dz,dzg,niter,rst,err
  Bus Assignment2 : BusAssignment  AssignedSignals=Ip,Wk,Wp,Wt,Wt0,Ft,Ft0,Vp,bp,bt,mu,li,bpli2,WN
  Bus Assignment3 : BusAssignment  AssignedSignals=cycle
  Bus Selector : BusSelector  OutputSignals=Ff,Bm,Ie,Ft,Ip,rBt
  Constant : Constant  Value=0  OutDataTypeStr=Bus: LYbus
  Cycle us : Subsystem
  Demux : Demux  Outputs=3
  FIR response matrix : Subsystem  Commented=on
  MEQINT : $bdroot/MEQINT  SystemSampleTime=-1
  MEQPOSTQ : Subsystem  Variant=on  VariantControl=Variant1
  Model Info : simulink/Model-Wide Utilities/Model Info  Frame=on  DisplayStringWithTags=|  HorizontalTextAlignment=Center  LeftAlignmentValue=0.5
      | Model Info
      | %<Creator>
      | %<ModifiedBy>
      | %<ModifiedDate>
      | %<ModifiedComment>
      | %<ModelVersion>
  Picard Iteration : Subsystem
  Reshape to match liut.m output : Reshape  OutputDimensionality=Customize  OutputDimensions=[L.nzx,L.nrx]
  Reshape to match liut.m output1 : Reshape  OutputDimensionality=Customize  OutputDimensions=[L.nzy,L.nry]
  Reshape to match liut.m output2 : Reshape  OutputDimensionality=Customize  OutputDimensions=[L.nzy,L.nry]
  To Workspace20 : ToWorkspace  VariableName=Bty  SampleTime=-1
  To Workspace7 : ToWorkspace  VariableName=Tdg  SampleTime=-1
  optional qint : Subsystem  Variant=on  VariantControl=Variant1
  t01/ Measurements : $bdroot/t01// Measurements  SystemSampleTime=-1
  LY : Outport
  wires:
  [zX] -> Bus Assignment/16
  [rX] -> Bus Assignment/15
  Picard Iteration/12(Out34) -> [zX]
  Picard Iteration/11(Out33) -> [rX]
  [nX] -> Bus Assignment/18
  Picard Iteration/14(Out32) -> [nX]
  [FX] -> Bus Assignment/17
  Bus Assignment2/1 -> optional qint/1("LY ")
  [Fx] -> optional qint/2(Fx)
  Picard Iteration/34(Out30) -> [Ff]
  Picard Iteration/33(Out29) -> [Bm]
  MEQINT/14 -> Bus Assignment2/15
  [iTQ] -> Bus Assignment/24
  Reshape to match liut.m output1/1 -> Bus Assignment/26
  [Iy] -> Reshape to match liut.m output1/1
  [Je] -> Bus Assignment/25
  Bus Selector/6 -> t01/ Measurements/6, [rBt]  "<rBt>"
  Bus Selector/4 -> t01/ Measurements/4  "<Ft>"
  [Opy] -> FIR response matrix/4(Opy)
  [FA] -> Bty/2
  [FA] -> FIR response matrix/2(FA)
  FIR response matrix/1(Tdg) -> To Workspace7/1
  [Opy] -> Bty/4
  [rBt] -> Bty/6
  Bty/1 -> To Workspace20/1
  [Fx] -> FIR response matrix/1(Fx)
  [ag] -> Bty/5
  [FB] -> FIR response matrix/3(FB)
  [Fx] -> Bty/1
  [FB] -> Bty/3
  [err] -> Bty/7
  Bus Assignment3/1 -> LY/1
  Cycle us/1(Out1) -> Bus Assignment3/2
  Reshape to match liut.m output/1 -> Bus Assignment/2
  MEQINT/13 -> Bus Assignment2/14
  Bus Assignment/1 -> Bus Assignment2/1
  [TQ] -> Bus Assignment/23
  [PQ] -> Bus Assignment/22
  [TTpQ] -> Bus Assignment/21
  [PpQ] -> Bus Assignment/20
  [lX] -> Bus Assignment/14
  [ag] -> Bus Assignment/19
  [nA] -> Bus Assignment/13
  [lB] -> Bus Assignment/12
  Picard Iteration/32(Out28) -> [lB]
  Picard Iteration/31(Out27) -> [nA]
  [Fx] -> Reshape to match liut.m output/1
  [rB] -> Bus Assignment/3
  [zB] -> Bus Assignment/4
  [FB] -> Bus Assignment/5
  [d2FA] -> Demux/1
  Demux/2 -> Bus Assignment/10
  Demux/3 -> Bus Assignment/11
  Demux/1 -> Bus Assignment/9
  [FA] -> Bus Assignment/8
  [zA] -> Bus Assignment/7
  [rA] -> Bus Assignment/6
  Picard Iteration/23(Out18) -> [iTQ]
  Picard Iteration/19(Out25) -> [PpQ]
  Picard Iteration/29(Out24) -> [dz]
  Picard Iteration/18(Out15) -> [Iy]
  Picard Iteration/5(Out6) -> [zA]
  Picard Iteration/30(Out4) -> [Je]
  Picard Iteration/20(Out26) -> [TTpQ]
  Picard Iteration/10(Out11) -> [FB]
  Picard Iteration/27(Out22) -> [ITpg]
  Picard Iteration/22(Out17) -> [TQ]
  Picard Iteration/17(Out14) -> [Opy]
  Picard Iteration/15(Out12) -> [lX]
  Picard Iteration/1(Out1) -> [rst]
  Picard Iteration/3(Out3) -> [niter]
  Picard Iteration/16(Out13) -> [Fx]
  Picard Iteration/28(Out23) -> [ag]
  Picard Iteration/26(Out21) -> [Tpg]
  Picard Iteration/25(Out20) -> [fTg]
  Picard Iteration/7(Out8) -> [d2FA]
  Picard Iteration/21(Out16) -> [PQ]
  Picard Iteration/2(Out2) -> [err]
  Picard Iteration/4(Out5) -> [rA]
  Picard Iteration/9(Out10) -> [zB]
  Picard Iteration/24(Out19) -> [fPg]
  Picard Iteration/6(Out7) -> [FA]
  Picard Iteration/8(Out9) -> [rB]
  Constant/1 -> Bus Assignment/1
  MEQINT/10 -> Bus Assignment2/11
  MEQINT/11 -> Bus Assignment2/12
  MEQINT/8 -> Bus Assignment2/9
  [ITpg] -> MEQINT/5
  MEQINT/4 -> Bus Assignment2/5
  [Tpg] -> MEQINT/4
  MEQINT/2 -> Bus Assignment2/3
  [Fx] -> MEQINT/6
  MEQINT/1 -> Bus Assignment2/2
  MEQINT/12 -> Bus Assignment2/13
  MEQINT/7 -> Bus Assignment2/8
  MEQINT/9 -> Bus Assignment2/10
  [rBt] -> MEQINT/8
  MEQINT/6 -> Bus Assignment2/7
  [fPg] -> MEQINT/2
  MEQINT/3 -> Bus Assignment2/4
  [fTg] -> MEQINT/3
  [Opy] -> MEQINT/7
  [ag] -> MEQINT/1
  MEQINT/5 -> Bus Assignment2/6
  t01/ Measurements/4 -> Picard Iteration/4(Ie)
  Bus Selector/3 -> t01/ Measurements/3  "<Ie>"
  Bus Selector/5 -> t01/ Measurements/5  "<Ip>"
  LX/1 -> Bus Selector/1
  BF parameters/1(" bfp") -> Picard Iteration/9(bfp)  "bfp"
  t01/ Measurements/8 -> Picard Iteration/8(sIp), [sIp]
  t01/ Measurements/7 -> Picard Iteration/7(FN)
  t01/ Measurements/6 -> Picard Iteration/6(rBt)
  t01/ Measurements/3 -> Picard Iteration/3(Yi)
  t01/ Measurements/2 -> Picard Iteration/2(Yd)
  Bus Selector/1 -> t01/ Measurements/1  "<Ff>"
  Bus Selector/2 -> t01/ Measurements/2  "<Bm>"
  t01/ Measurements/1 -> Picard Iteration/1(Yr)
  optional qint/1(" LYo") -> MEQPOSTQ/1("LY ")
  [sIp] -> MEQPOSTQ/2("sIp ")
  MEQPOSTQ/1(" LYo") -> Bus Assignment3/1
  [Bm] -> Bus Assignment/28
  [rBt] -> Bus Assignment/30
  [Ff] -> Bus Assignment/29
  [dz] -> Bus Assignment/31
  [dz] -> Bus Assignment/32
  [niter] -> Bus Assignment/33
  [rst] -> Bus Assignment/34
  [err] -> Bus Assignment/35
  [Opy] -> Reshape to match liut.m output2/1
  Reshape to match liut.m output2/1 -> Bus Assignment/27
  t01/ Measurements/5 -> Picard Iteration/5(Ip)
  Picard Iteration/13(Out31) -> [FX]

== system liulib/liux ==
  Bm1 : FromWorkspace  VariableName=struct('time',[],'signals',struct('values',single(LX.Bm')))  SampleTime=L.dt  Interpolate=off  OutputAfterFinalValue=Holding final value
  Bus Assignment : BusAssignment  AssignedSignals=Ff,Bm,Ie,Ft,Ip,rBt
  Constant : Constant  Value=0  OutDataTypeStr=Bus: LXbus
  Ff1 : FromWorkspace  VariableName=struct('time',[],'signals',struct('values',single(LX.Ff')))  SampleTime=L.dt  Interpolate=off  OutputAfterFinalValue=Holding final value
  Ft1 : FromWorkspace  VariableName=struct('time',[],'signals',struct('values',single(LX.Ft')))  SampleTime=L.dt  Interpolate=off  OutputAfterFinalValue=Holding final value
  Ft2 : FromWorkspace  VariableName=struct('time',[],'signals',struct('values',single(LX.Ip')))  SampleTime=L.dt  Interpolate=off  OutputAfterFinalValue=Holding final value
  Ia1 : FromWorkspace  VariableName=struct('time',[],'signals',struct('values',single(LX.Ie')))  SampleTime=L.dt  Interpolate=off  OutputAfterFinalValue=Holding final value
  RBt1 : FromWorkspace  VariableName=struct('time',[],'signals',struct('values',single(LX.rBt')))  SampleTime=L.dt  Interpolate=off  OutputAfterFinalValue=Holding final value
  LX : Outport  OutDataTypeStr=Bus: LXbus
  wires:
  Constant/1 -> Bus Assignment/1
  Bus Assignment/1 -> LX/1
  Ft2/1 -> Bus Assignment/6  "Ip"
  RBt1/1 -> Bus Assignment/7  "rBt"
  Ft1/1 -> Bus Assignment/5  "Ft"
  Ia1/1 -> Bus Assignment/4  "Ia"
  Bm1/1 -> Bus Assignment/3  "Bm"
  Ff1/1 -> Bus Assignment/2  "Ff"

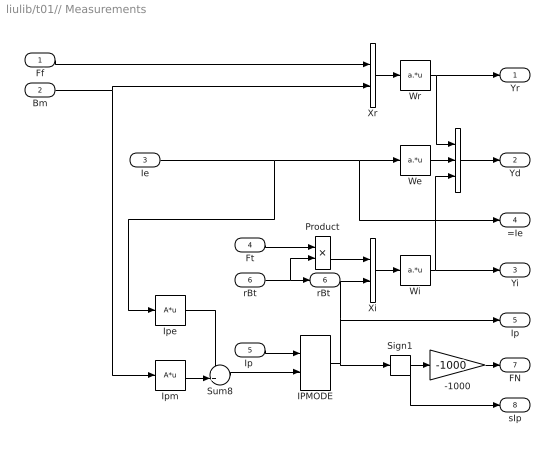
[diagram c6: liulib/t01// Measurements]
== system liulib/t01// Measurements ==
  Ff : Inport
  Bm : Inport  Port=2
  Ie : Inport  Port=3
  Ft : Inport  Port=4
  "Ip " : Inport  Port=5
  rBt : Inport  Port=6
  " " : Concatenate  NumInputs=3
  -1000 : Gain  Gain=-1000
  IPMODE : VariantSource
  Ipe : mkllib/A*u  A=single([L.Ipa L.Ipu])
  Ipm : mkllib/A*u  A=single(L.G.Ipm)
  Product : Product
  Sign1 : Signum
  Sum8 : Sum  Inputs=++|
  We : mkllib/a.*u  a=single(L.We)
  Wi : mkllib/a.*u  a=single(L.Wi)
  Wr : mkllib/a.*u  a=single(L.Wr)
  Xi : Concatenate
  Xr : Concatenate
  Yr : Outport
  Yd : Outport  Port=2
  Yi : Outport  Port=3
  =Ie : Outport  Port=4
  Ip : Outport  Port=5
  "rBt " : Outport  Port=6
  FN : Outport  Port=7
  sIp : Outport  Port=8
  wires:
  " "/1 -> Yd/1
  We/1 -> " "/2
  Wi/1 -> Yi/1, " "/3
  Wr/1 -> Yr/1, " "/1
  Xi/1 -> Wi/1
  Xr/1 -> Wr/1
  Product/1 -> Xi/1
  Ft/1 -> Product/1
  rBt/1 -> Product/2, "rBt "/1
  IPMODE/1 -> Ip/1, Xi/2, Sign1/1
  Sign1/1 -> sIp/1, -1000/1
  -1000/1 -> FN/1
  Ipm/1 -> Sum8/2
  Ipe/1 -> Sum8/1
  "Ip "/1 -> IPMODE/1
  Sum8/1 -> IPMODE/2
  Ff/1 -> Xr/1
  Ie/1 -> Ipe/1, We/1, =Ie/1
  Bm/1 -> Xr/2, Ipm/1

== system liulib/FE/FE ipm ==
  Yd : Inport
  Ie : Inport  Port=2
  Ip : Inport  Port=3
  sIp : Inport  Port=4
  1/nh : Constant  Value=repmat(single(1/L.nh),L.nh,1)  OutDataTypeStr=single
  Divide : Product  Inputs=**
  Divide1 : Product  Inputs=***
  IPMH : $bdroot/IPMH  Ahd=L.Ahd  Aed=L.Aed  Ahe=L.Ahe  Aeh=L.Aeh  Ahh=L.Ahh  uAhh=L.uAhh  nit=L.P.iterh
  Terminator1 : Terminator
  tolh/nh : Constant  Value=single(L.P.tolh/L.nh)  OutDataTypeStr=single
  Jh : Outport
  Je : Outport  Port=2
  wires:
  Ip/1 -> Divide1/2, Divide/1
  Yd/1 -> IPMH/1
  Ie/1 -> IPMH/2
  sIp/1 -> IPMH/4, Divide1/1
  IPMH/2 -> Jh/1
  IPMH/1 -> Je/1
  IPMH/3 -> Terminator1/1
  1/nh/1 -> Divide/2
  Divide1/1 -> IPMH/5
  Divide/1 -> IPMH/3
  tolh/nh/1 -> Divide1/3

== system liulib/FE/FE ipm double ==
  Yd : Inport
  Ie : Inport  Port=2
  Ip : Inport  Port=3
  sIp : Inport  Port=4
  1/nh : Constant  Value=repmat(1/L.nh,L.nh,1)  OutDataTypeStr=double
  Data Type Conversion{,1..3} (4 alike) : DataTypeConversion  OutDataTypeStr=double
  Data Type Conversion4 : DataTypeConversion  OutDataTypeStr=single
  Data Type Conversion5 : DataTypeConversion  OutDataTypeStr=single
  Divide : Product  Inputs=**
  Divide1 : Product  Inputs=***
  Terminator1 : Terminator
  dIPMH : $bdroot/dIPMH  Ahd=double(L.Ahd)  Aed=double(L.Aed)  Ahe=double(L.Ahe)  Aeh=double(L.Aeh)  Ahh=double(L.Ahh)  uAhh=double(L.uAhh)  nit=L.P.iterh
  tolh/nh : Constant  Value=L.P.tolh/L.nh  OutDataTypeStr=double
  Jh : Outport
  Je : Outport  Port=2
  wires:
  Ie/1 -> Data Type Conversion1/1
  1/nh/1 -> Divide/2
  Divide/1 -> dIPMH/3
  sIp/1 -> Data Type Conversion3/1
  dIPMH/1 -> Data Type Conversion4/1
  dIPMH/3 -> Terminator1/1
  tolh/nh/1 -> Divide1/3
  Divide1/1 -> dIPMH/5
  dIPMH/2 -> Data Type Conversion5/1
  Ip/1 -> Data Type Conversion2/1
  Yd/1 -> Data Type Conversion/1
  Data Type Conversion/1 -> dIPMH/1
  Data Type Conversion1/1 -> dIPMH/2
  Data Type Conversion2/1 -> Divide1/2, Divide/1
  Data Type Conversion3/1 -> dIPMH/4, Divide1/1
  Data Type Conversion4/1 -> Je/1
  Data Type Conversion5/1 -> Jh/1

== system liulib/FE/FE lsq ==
  Yd : Inport
  Ie : Inport  Port=2
  Ip : Inport  Port=3
  sIp : Inport  Port=4
  Aed : mkllib/A*u  A=L.Aed
  Ahd : mkllib/A*u  A=L.Ahd
  Terminator : Terminator
  Terminator1 : Terminator
  Terminator2 : Terminator
  Jh : Outport
  Je : Outport  Port=2
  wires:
  Ahd/1 -> Jh/1
  Yd/1 -> Aed/1, Ahd/1
  Aed/1 -> Je/1
  Ie/1 -> Terminator/1
  Ip/1 -> Terminator1/1
  sIp/1 -> Terminator2/1

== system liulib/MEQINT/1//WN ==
  note: WN=(\mu_0 I_p^2)/4
  Ip : Inport
  1./u : mkllib/1.//u
  Constant1 : Constant  Value=0  OutDataTypeStr=single
  Constant2 : Constant  Value=single(1/(1e-7*pi*L.P.r0))  OutDataTypeStr=single
  Product1 : Product  Inputs=*/
  Product2 : Product
  Switch : Switch  Criteria=u2 ~= 0
  WN : Outport
  1/WN : Outport  Port=2
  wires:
  1./u/1 -> Switch/1
  Product1/1 -> WN/1, 1./u/1
  Ip/1 -> Switch/2, Product2/2, Product2/1
  Constant2/1 -> Product1/2
  Product2/1 -> Product1/1
  Switch/1 -> 1/WN/1
  Constant1/1 -> Switch/3

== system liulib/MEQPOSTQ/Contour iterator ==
  rst : Inport
  rA : Inport  Port=2
  zA : Inport  Port=3
  FA : Inport  Port=4
  FB : Inport  Port=5
  Fx : Inport  Port=6
  Opy : Inport  Port=7
  Flux contours : Subsystem  TreatAsAtomicUnit=on
  For Iterator : ForIterator  IterationLimit=L.P.iterq  ShowIterationPort=off
  Unit Delay : UnitDelay  SampleTime=-1  HasFrameUpgradeWarning=on
  aq : Outport
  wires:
  rst/1 -> Flux contours/2(rst)
  rA/1 -> Flux contours/3(rA)
  zA/1 -> Flux contours/4(zA)
  Unit Delay/1 -> Flux contours/1(zaq)
  Fx/1 -> Flux contours/7(Fx)
  FA/1 -> Flux contours/5(FA)
  FB/1 -> Flux contours/6(FB)
  Flux contours/1(aq) -> Unit Delay/1, aq/1
  Opy/1 -> Flux contours/8(Opy)

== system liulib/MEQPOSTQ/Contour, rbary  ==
  rq : Inport
  zq : Inport  Port=2
  Divide : Product  Inputs=*/
  Dot Product : DotProduct
  Gain : Gain  Gain=1/2
  Product : Product
  Product1 : Product
  Selector4 : Selector  NumberOfDimensions=2  IndexOptions=Index vector (dialog),Select all  Indices=[2:L.noq,1],1  OutputSizes=1,1
  Selector5 : Selector  NumberOfDimensions=2  IndexOptions=Index vector (dialog),Select all  Indices=[2:L.noq,1],1  OutputSizes=1,1
  Sqrt1 : Sqrt
  Subtract : Sum  Inputs=+-
  Subtract1 : Sum  Inputs=+-
  Subtract2 : Sum
  Subtract3 : Sum
  Sum of Elements : Sum  Inputs=+
  rbary : Outport
  Lp : Outport  Port=2
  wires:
  Divide/1 -> rbary/1  "rbary"
  zq/1 -> Selector5/1, Subtract1/2
  rq/1 -> Selector4/1, Subtract/2, Subtract3/2
  Subtract/1 -> Product/1, Product/2
  Subtract2/1 -> Sqrt1/1
  Sum of Elements/1 -> Lp/1, Divide/2  "Lp"
  Subtract3/1 -> Gain/1
  Gain/1 -> Dot Product/1  "R(q) trapezoidal"
  Selector4/1 -> Subtract/1, Subtract3/1
  Product/1 -> Subtract2/1
  Selector5/1 -> Subtract1/1
  Subtract1/1 -> Product1/1, Product1/2
  Product1/1 -> Subtract2/2
  Dot Product/1 -> Divide/1
  Sqrt1/1 -> Dot Product/2, Sum of Elements/1  "dq"

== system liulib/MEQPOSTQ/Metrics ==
  aq : Inport
  rst : Inport  Port=2
  *M1q : mkllib/U*A  A=L.M1q
  Constant : Constant  Value=zeros(L.noq,L.npq)  OutDataTypeStr=single
  Coq : Product  Inputs=/*
  M2q* : mkllib/A*U  A=L.M2q
  Product : Product
  Product2 : Product  Inputs=/**
  Switch : Switch  Criteria=u2 > Threshold
  Switch1 : Switch  Criteria=u2 > Threshold
  qaq1 : Sum  Inputs=|++
  da^2/pdp = M1q : Outport
  ((da^2/2do)^2+a^2)/(da^2/pdp) = M2q : Outport  Port=2
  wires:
  aq/1 -> Product/1, Product/2
  Product/1 -> *M1q/1, M2q*/1, Product2/1, qaq1/1
  *M1q/1 -> Coq/1, Switch/3
  M2q*/1 -> Product2/2, Product2/3
  Product2/1 -> qaq1/2
  qaq1/1 -> Coq/2
  Coq/1 -> Switch1/3
  Switch/1 -> da^2/pdp = M1q/1
  rst/1 -> Switch1/2, Switch/2
  Constant/1 -> Switch1/1, Switch/1
  Switch1/1 -> ((da^2/2do)^2+a^2)/(da^2/pdp) = M2q/1

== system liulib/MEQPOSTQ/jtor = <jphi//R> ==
  PpQ : Inport
  TTpQ : Inport  Port=2
  Q2Q : Inport  Port=3
  Add : Sum
  Gain : Gain  Gain=single(2*pi*L.P.r0)
  Gain1 : Gain  Gain=single(1/(4e-7*pi))
  Product : Product
  jtorQ : Outport
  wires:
  TTpQ/1 -> Product/1
  PpQ/1 -> Add/1
  Q2Q/1 -> Product/2
  Gain/1 -> jtorQ/1
  Product/1 -> Gain1/1
  Add/1 -> Gain/1
  Gain1/1 -> Add/2

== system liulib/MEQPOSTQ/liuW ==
  LY : Inport
  dummy : Subsystem  VariantControl=liuAWMODEvariant0
  liuW : Subsystem  VariantControl=liuAWMODEvariant1
  LYo : Outport

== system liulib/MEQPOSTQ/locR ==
  LY : Inport
  "raQ " : Inport  Port=2
  "qQ " : Inport  Port=3
  sq : Inport  Port=4
  dummy : Subsystem  VariantControl=liuLOCRMODEvariant0
  locR : Subsystem  VariantControl=liuLOCRMODEvariant1
  " LYo" : Outport

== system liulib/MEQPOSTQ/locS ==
  "LY " : Inport
  dummy : Subsystem  VariantControl=liuLOCSMODEvariant0
  locS : Subsystem  VariantControl=liuLOCSMODEvariant1
  " LYo" : Outport

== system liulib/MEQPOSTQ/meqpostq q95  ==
  iqQ : Inport
  1./u : mkllib/1.//u
  Gain : Gain  Gain=L.c95  Multiplication=Matrix(K*u) (u vector)
  Selector4 : Selector  IndexOptions=Index vector (dialog)  Indices=L.i95  OutputSizes=1
  q95 : Outport
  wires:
  Gain/1 -> 1./u/1
  iqQ/1 -> Selector4/1
  Selector4/1 -> Gain/1
  1./u/1 -> q95/1

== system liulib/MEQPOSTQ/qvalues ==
  aq : Inport
  iqQ : Inport  Port=2
  sq : Inport  Port=3
  1/U : mkllib/1//U
  Constant4 : Constant  Value=L.raN  OutDataTypeStr=single
  Gain : Gain  Gain=-1
  Normalized Radius : Subsystem
  minQ : $bdroot/minQ  nmin=1
  raQ : Outport
  raqmin : Outport  Port=2
  qmin : Outport  Port=3
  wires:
  1/U/1 -> qmin/1
  Constant4/1 -> minQ/4
  minQ/1 -> raqmin/1
  minQ/2 -> 1/U/1
  sq/1 -> Gain/1
  Normalized Radius/1(raQ) -> minQ/1, raQ/1
  aq/1 -> Normalized Radius/1(aq)
  iqQ/1 -> minQ/2
  Gain/1 -> minQ/3

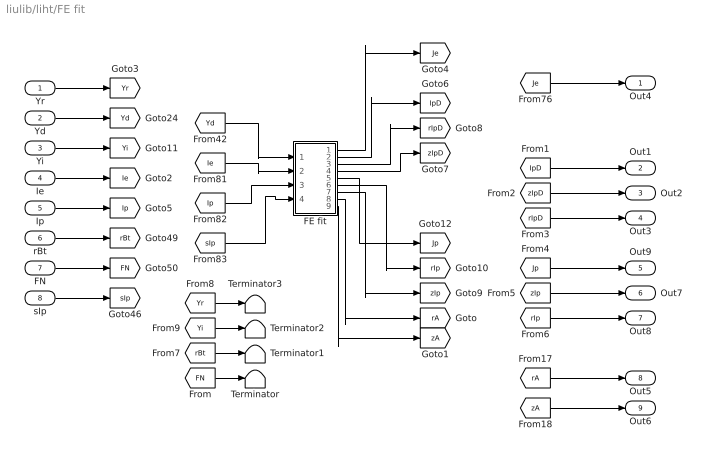
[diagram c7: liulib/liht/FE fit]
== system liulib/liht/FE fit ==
  Yr : Inport
  Yd : Inport  Port=2
  Yi : Inport  Port=3
  Ie : Inport  Port=4
  Ip : Inport  Port=5
  rBt : Inport  Port=6
  FN : Inport  Port=7
  sIp : Inport  Port=8
  FE fit : Subsystem
  Terminator{,1..3} (4 alike) : Terminator
  Out4 : Outport
  Out1 : Outport  Port=2
  Out2 : Outport  Port=3
  Out3 : Outport  Port=4
  Out9 : Outport  Port=5
  Out7 : Outport  Port=6
  Out8 : Outport  Port=7
  Out5 : Outport  Port=8
  Out6 : Outport  Port=9
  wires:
  FE fit/9(zA) -> [zA]
  FE fit/8(rA) -> [rA]
  rBt/1 -> [rBt]
  FN/1 -> [FN]
  sIp/1 -> [sIp]
  Yr/1 -> [Yr]
  Yi/1 -> [Yi]
  Ip/1 -> [Ip]
  Yd/1 -> [Yd]
  Ie/1 -> [Ie]
  [zA] -> Out6/1
  [rA] -> Out5/1
  [Je] -> Out4/1
  [Yd] -> FE fit/1(Yd)
  [Ie] -> FE fit/2(Ie)
  [Ip] -> FE fit/3(Ip_in)
  [sIp] -> FE fit/4(sIp)
  FE fit/1(Je) -> [Je]
  FE fit/5(Ip) -> [Jp]
  FE fit/7(zIp) -> [zIp]
  FE fit/6(rIp) -> [rIp]
  FE fit/3(rIpD) -> [rIpD]
  FE fit/4(zIpD) -> [zIpD]
  FE fit/2(IpD) -> [IpD]
  [IpD] -> Out1/1
  [zIpD] -> Out2/1
  [rIpD] -> Out3/1
  [zIp] -> Out7/1
  [rIp] -> Out8/1
  [Jp] -> Out9/1
  [FN] -> Terminator/1
  [rBt] -> Terminator1/1
  [Yi] -> Terminator2/1
  [Yr] -> Terminator3/1

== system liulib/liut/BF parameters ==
  BF3I : Subsystem  VariantControl=liuBFCTMODEvariant2
  BF3P : Subsystem  VariantControl=liuBFCTMODEvariant1
  BFEF : Subsystem  VariantControl=liuBFCTMODEvariant3
  " bfp" : Outport

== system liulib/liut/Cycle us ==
  Data Type Conversion : DataTypeConversion
  Memory : Memory  InheritSampleTime=on
  Sum : Sum  Inputs=|+-
  Wall time : $bdroot/Wall time  f=1000000
  Out1 : Outport  OutDataTypeStr=single
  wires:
  Data Type Conversion/1 -> Out1/1
  Memory/1 -> Sum/2, Wall time/1
  Sum/1 -> Data Type Conversion/1
  Wall time/1 -> Memory/1, Sum/1

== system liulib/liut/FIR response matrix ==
  Fx : Inport
  FA : Inport  Port=2
  FB : Inport  Port=3
  Opy : Inport  Port=4
  BF3I4 : $bdroot/BF3I4  nzy=L.nzy  nry=L.nry
  Constant : Constant  Value=ones(21,3)  VectorParams1D=off  OutDataTypeStr=single
  Constant1 : Constant  Value=0:9  OutDataTypeStr=uint32
  Constant2 : Constant  Value=[ones(10,1) zeros(10,1)]  OutDataTypeStr=single
  Terminator : Terminator
  Tdg : Outport
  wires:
  FB/1 -> BF3I4/3
  BF3I4/1 -> Tdg/1
  Constant/1 -> BF3I4/5
  Constant1/1 -> BF3I4/6
  FA/1 -> BF3I4/2
  Constant2/1 -> BF3I4/7
  Opy/1 -> BF3I4/4
  Fx/1 -> BF3I4/1
  BF3I4/2 -> Terminator/1

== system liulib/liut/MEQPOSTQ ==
  "LY " : Inport
  "sIp " : Inport  Port=2
  Direct pass : Subsystem  VariantControl=liuITERQMODEvariant0
  MEQPOSTQ : $bdroot/MEQPOSTQ  SystemSampleTime=-1  VariantControl=liuITERQMODEvariant1
  " LYo" : Outport
